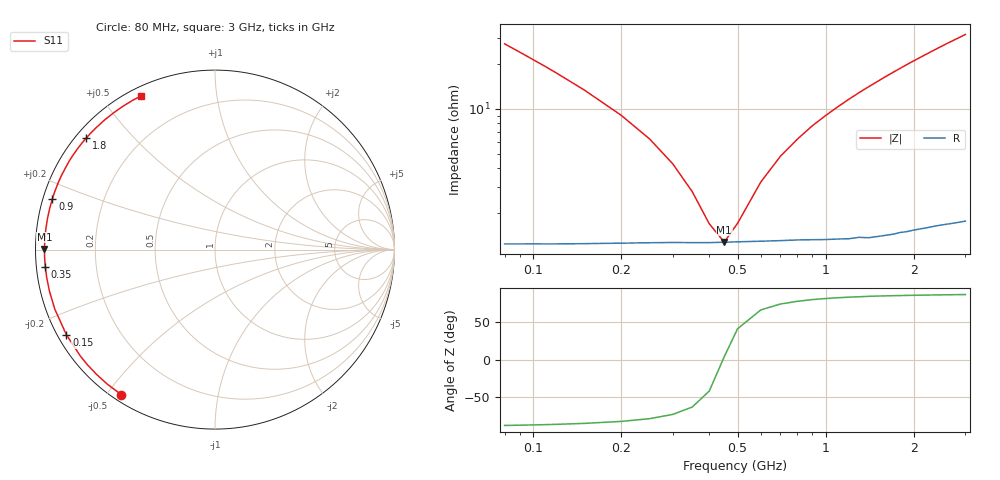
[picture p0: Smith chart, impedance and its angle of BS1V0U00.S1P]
! SIEMENS Small Signal Semiconductors
! BB640
! Si Tuning Diode in SOD323
! VR = 1 V
! S-Parameters:  July  1993
# GHz  S  MA  R  50
!  f  S11
! GHz  MAG  ANG
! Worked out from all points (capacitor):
!   33 points, 80 MHz to 3 GHz, reference 50 ohm
!   read as one part to ground: C = 70.7 pF near 80 MHz
!   lowest |Z| = 1.29 ohm at 450 MHz (marker M1)
!   series resonance near 446.4 MHz, so ESL is about 1.8 nH
!   S11 on the Smith chart (normalised r, x): 80 MHz: 0.02, -0.54; 150 MHz: 0.03, -0.27; 350 MHz: 0.03, -0.05; 900 MHz: 0.03, +0.15; 1.8 GHz: 0.03, +0.37; 3 GHz: 0.04, +0.63
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0.08  0.9622 -122.8
0.09  0.9602 -128.7
0.1  0.9586 -133.7
0.11  0.9574 -137.9
0.12  0.9564 -141.6
0.15  0.9542 -150.2
0.2  0.9522 -159.6
0.25  0.9511 -165.9
0.3  0.9505 -170.6
0.35  0.9504 -174.3
0.4  0.9503 -177.4
0.45  0.95 179.8
0.5  0.9497 177.4
0.6  0.9494 173.2
0.7  0.9492 169.4
0.9  0.9492 162.7
1  0.9495 159.7
1.2  0.9499 154.0
1.4  0.9503 148.7
1.6  0.9498 143.7
1.7  0.9496 141.3
1.8  0.949 139.0
2  0.9487 134.5
2.2  0.9487 130.3
2.4  0.9487 126.3
2.6  0.9492 122.5
2.8  0.9498 119.0
3  0.9504 115.6
